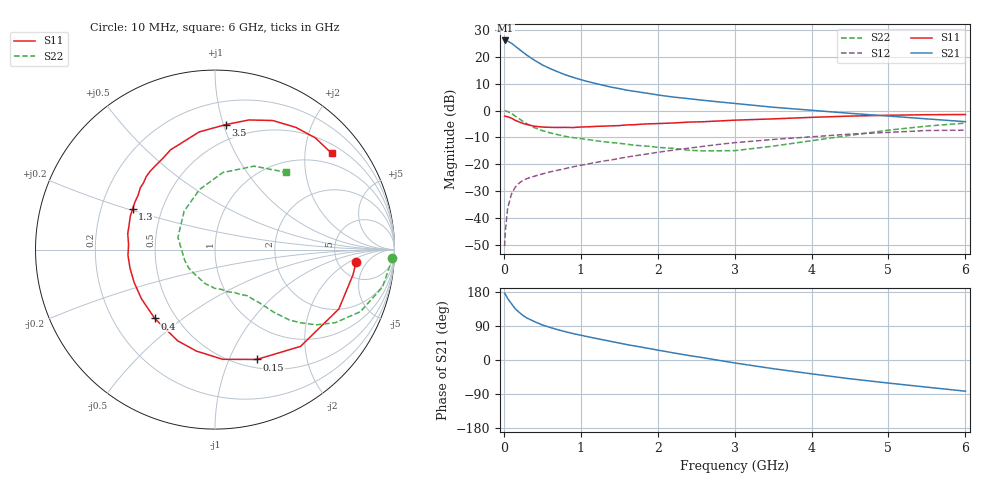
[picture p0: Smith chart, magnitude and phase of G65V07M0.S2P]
! SIEMENS Small Signal Semiconductors
! BFG193
! Si NPN RF Bipolar Junction Transistor in SOT223
! VCE = 5 V  IC = 7 mA
! Common Emitter S-Parameters:  August  1996
# GHz  S  MA  R  50
!  f  S11  S21  S12  S22
! GHz  MAG  ANG  MAG  ANG  MAG  ANG  MAG  ANG
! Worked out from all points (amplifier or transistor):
!   36 points, 10 MHz to 6 GHz, reference 50 ohm
!   highest |S21| = 26.1 dB at 20 MHz (marker M1)
!   |S21| within 3 dB of that: start of sweep to 187 MHz
!   unconditionally stable (mu >= 1): 1.034 GHz to 2.557 GHz
!   at 250 MHz: K = 0.42, MSG = 23.8 dB, |S12| = -26.0 dB
!   at 1.4 GHz: K = 1.08, MAG = 11.8 dB, |S12| = -18.4 dB
!   at 6 GHz: K = 0.86, MSG = 1.6 dB, |S12| = -7.3 dB
!   S11 on the Smith chart (normalised r, x): 10 MHz: 7.39, -2.80; 150 MHz: 0.59, -1.27; 400 MHz: 0.38, -0.40; 1.3 GHz: 0.34, +0.21; 3.5 GHz: 0.37, +1.02; 6 GHz: 0.71, +2.61
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0.01  0.7887 -5.2  20.09 176.2  0.003 95.3  0.9876 -2.6
0.02  0.7815 -10.4  20.1 173.5  0.0058 84.8  0.9791 -5.1
0.05  0.7652 -25.6  19.49 162.2  0.0155 78.0  0.9563 -12.6
0.1  0.7198 -48.5  17.82 148.4  0.0281 67.7  0.881 -23.1
0.15  0.6549 -69.1  15.64 134.9  0.038 58.6  0.7838 -31.3
0.2  0.6128 -86.0  13.77 125.6  0.0448 53.9  0.7028 -36.6
0.25  0.5748 -100.4  12.1 117.4  0.0503 49.8  0.6246 -40.7
0.3  0.5492 -112.2  10.7 110.8  0.0541 47.9  0.5682 -43.5
0.4  0.5098 -131.2  8.574 101.1  0.0602 45.4  0.4787 -46.8
0.5  0.4929 -146.3  7.055 92.5  0.0662 44.0  0.4226 -48.6
0.6  0.4863 -157.9  6.037 86.0  0.0722 44.0  0.3847 -50.2
0.7  0.4847 -167.5  5.261 80.0  0.0774 44.6  0.3558 -52.1
0.9  0.4823 176.7  4.142 69.8  0.0898 44.7  0.3134 -55.1
1.1  0.4975 164.4  3.43 61.1  0.1018 44.7  0.2871 -60.5
1.3  0.512 153.8  2.928 52.8  0.1153 44.1  0.2624 -65.5
1.6  0.5399 140.4  2.39 40.6  0.1362 41.6  0.2367 -76.6
2.2  0.5856 119.7  1.782 19.0  0.1833 34.1  0.1982 -105.4
2.8  0.6398 102.4  1.445 -1.1  0.2349 23.9  0.1787 -145.4
3.5  0.699 85.1  1.152 -22.9  0.2897 8.7  0.2176 161.8
4.5  0.7879 65.9  0.887 -49.5  0.3646 -11.4  0.3457 104.4
5.5  0.8364 48.1  0.699 -71.7  0.4243 -36.6  0.5134 64.9
6  0.8425 39.6  0.62 -82.3  0.432 -51.1  0.5836 47.6
